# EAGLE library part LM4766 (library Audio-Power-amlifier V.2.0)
LM4766 Overture™ Audio Power Amplifier Series Dual 40W Audio Power Amplifier with Mute
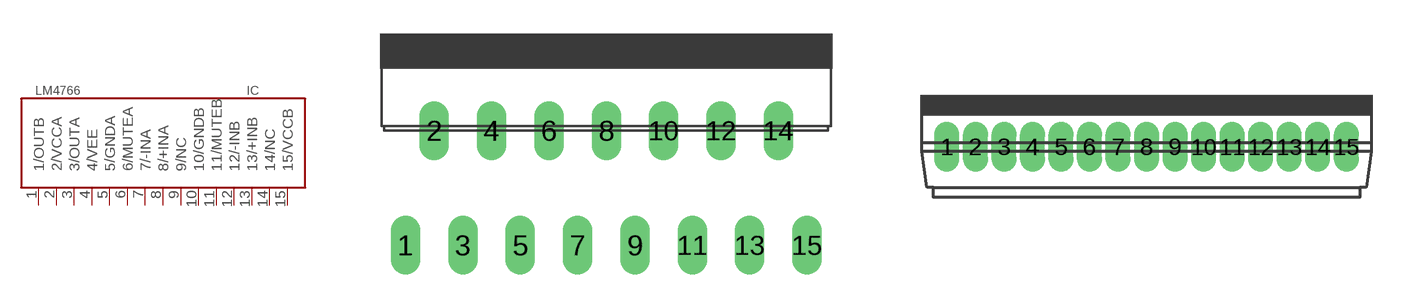
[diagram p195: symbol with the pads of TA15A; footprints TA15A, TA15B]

Designator prefix IC

## LM4766LM4766T/LF15  [TA15A]
1  1/OUTB  out
2  2/VCCA  pwr
3  3/OUTA  out
4  4/VEE  pwr
5  5/GNDA  pwr
6  6/MUTEA  in
7  7/-INA  in
8  8/+INA  in
9  9/NC  nc
10  10/GNDB  pwr
11  11/MUTEB  in
12  12/-INB  in
13  13/+INB  in
14  14/NC  nc
15  15/VCCB  pwr

## LM4766LM4766T/NOPB  [TA15B]
Pads as for TA15A

## LM4766LM4766TF/NOPB  [TF15A]
Pads as for TA15A

## Footprint TA15A (pad centres in mm)
TA15A www.national.com
drill 0.8 long: 1 -8.89,-5.08; 2 -7.62,0; 3 -6.35,-5.08; 4 -5.08,0; 5 -3.81,-5.08; 6 -2.54,0; 7 -1.27,-5.08; 8 0,0; 9 1.27,-5.08; 10 2.54,0; 11 3.81,-5.08; 12 5.08,0; 13 6.35,-5.08; 14 7.62,0; 15 8.89,-5.08

## Footprint TA15B (pad centres in mm)
TA15B
drill 0.6 pad 1.016 long: 1 -8.89,0; 2 -7.62,0; 3 -6.35,0; 4 -5.08,0; 5 -3.81,0; 6 -2.54,0; 7 -1.27,0; 8 0,0; 9 1.27,0; 10 2.54,0; 11 3.81,0; 12 5.08,0; 13 6.35,0; 14 7.62,0; 15 8.89,0

## Footprint TF15A (pad centres in mm)
TF15A www.national.com
drill 0.8 long: 1 -8.89,-5.08; 2 -7.62,0; 3 -6.35,-5.08; 4 -5.08,0; 5 -3.81,-5.08; 6 -2.54,0; 7 -1.27,-5.08; 8 0,0; 9 1.27,-5.08; 10 2.54,0; 11 3.81,-5.08; 12 5.08,0; 13 6.35,-5.08; 14 7.62,0; 15 8.89,-5.08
